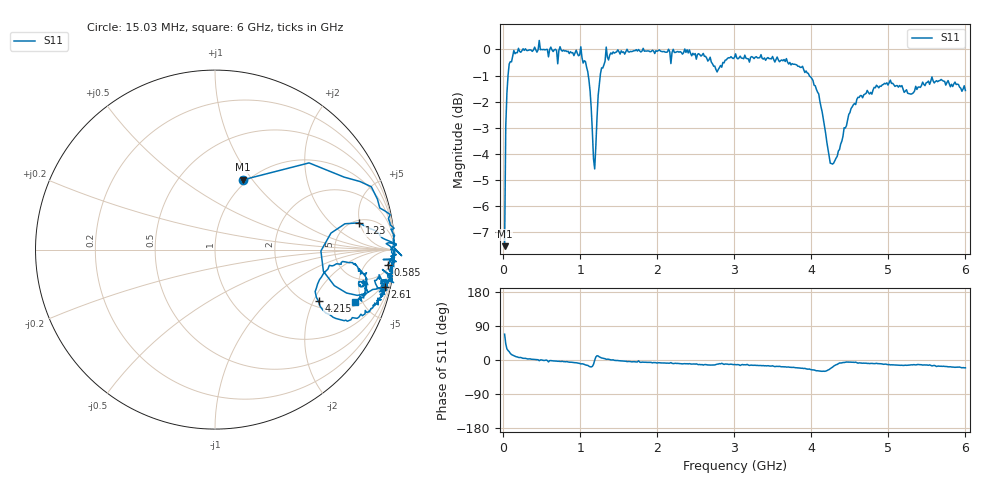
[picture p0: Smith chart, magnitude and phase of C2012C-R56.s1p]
!	Network	Analyzer	HP8753E.07.74:	Oct	30	2002	Serial	No.	JP38451487
!	Hewlett-Packard
!	28	Aug	2009	12:43:39
!	Frequency	S11
#	HZ	S	RI	R	50
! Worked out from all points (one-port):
!   400 points, 15.03 MHz to 6 GHz, reference 50 ohm
!   lowest |S11| = -7.5 dB at 15.03 MHz (marker M1), VSWR 2.45, Z = 47.8 + j45.1 ohm
!   |S11| at or under -10 dB: nowhere
!   S11 on the Smith chart (normalised r, x): 15.03 MHz: 0.96, +0.90; 585 MHz: 7, -20; 1.23 GHz: 5.45, +4.85; 2.61 GHz: 1.30, -9.13; 4.215 GHz: 2.23, -2.20; 6 GHz: 2.27, -4.38
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1.502992e7  0.157 0.389
3.002985e7  0.524 0.483
4.502978e7  0.719 0.404
7.502962e7  0.871 0.35
1.350293e8  0.976 0.195
4.650277e8  1.04 -0.0341
5.550272e8  1 -0.000732
5.850271e8  0.964 -0.085
7.650262e8  0.991 -0.0566
1.005025e9  0.995 -0.184
1.125024e9  0.793 -0.255
1.155024e9  0.665 -0.201
1.185024e9  0.59 -0.00751
1.230024e9  0.802 0.149
1.335023e9  1.01 0.0315
1.515022e9  0.979 -0.0372
2.265019e9  0.979 -0.155
2.610017e9  0.948 -0.206
2.835016e9  0.914 -0.14
3.015015e9  0.958 -0.21
3.765011e9  0.884 -0.31
4.06501e9  0.737 -0.399
4.215009e9  0.577 -0.288
4.365008e9  0.637 -0.0877
4.515007e9  0.767 -0.0727
4.845006e9  0.844 -0.129
5.265004e9  0.8 -0.193
6e9  0.781 -0.293
